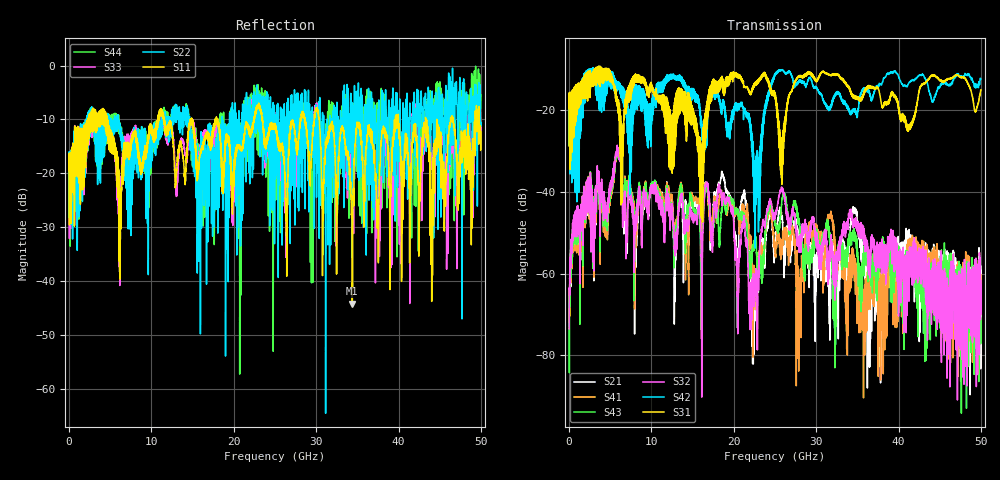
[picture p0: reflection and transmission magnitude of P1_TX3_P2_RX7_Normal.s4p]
!Keysight Technologies,N5225B,MY57041031,A.13.20.10
!Date: Friday, May 31, 2019 11:38:36
!Correction: S11(Full 4 Port(1,2,3,4))
!S12(Full 4 Port(1,2,3,4))
!S13(Full 4 Port(1,2,3,4))
!S14(Full 4 Port(1,2,3,4))
!S21(Full 4 Port(1,2,3,4))
!S22(Full 4 Port(1,2,3,4))
!S23(Full 4 Port(1,2,3,4))
!S24(Full 4 Port(1,2,3,4))
!S31(Full 4 Port(1,2,3,4))
!S32(Full 4 Port(1,2,3,4))
!S33(Full 4 Port(1,2,3,4))
!S34(Full 4 Port(1,2,3,4))
!S41(Full 4 Port(1,2,3,4))
!S42(Full 4 Port(1,2,3,4))
!S43(Full 4 Port(1,2,3,4))
!S44(Full 4 Port(1,2,3,4))
!S4P File: Measurements: <S11,S12,S13,S14>,
!<S21,S22,S23,S24>,
!<S31,S32,S33,S34>,
!<S41,S42,S43,S44>:
# Hz S  dB  R 50.0
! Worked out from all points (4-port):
!   5000 points, 10 MHz to 50 GHz, reference 50 ohm
!   strongest paths, dB at 10 MHz, 12.51 GHz, 25.01 GHz, 37.51 GHz, 50 GHz:
!     S31: -19.5, -27.1, -15.7, -14.5, -15.0
!     S42: -19.4, -12.2, -11.6, -14.0, -12.4
!     S32: -73.5, -42.8, -45.8, -55.0, -69.5
!     S43: -65.2, -42.9, -47.9, -57.0, -70.8
!     S41: -71.1, -40.8, -54.3, -69.6, -68.4
!     S21: -67.7, -41.2, -53.6, -64.7, -58.1
!   lowest |S11| = -44.2 dB at 34.39 GHz (marker M1), VSWR 1.01, Z = 50 + j0.617 ohm
!   |S11| at or under -10 dB: 4.66 GHz to 10.77 GHz (6.106 GHz wide, 79.2 % of centre); 23.49 GHz to 28.08 GHz (4.584 GHz wide, 17.8 % of centre); 30.37 GHz to 39.61 GHz (9.24 GHz wide, 26.4 % of centre)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
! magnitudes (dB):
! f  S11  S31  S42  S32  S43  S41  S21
! 10 MHz  -19.5  -19.5  -19.4  -73.5  -65.2  -71.1  -67.7
! 6.05 GHz  -29.4  -18.9  -14.4  -31.7  -31.4  -31.4  -31.4
! 21.24 GHz  -13.9  -14.2  -20.0  -46.3  -46.5  -45.4  -39.8
! 22.43 GHz  -10.2  -13.7  -35.1  -63.9  -52.8  -61.6  -72.5
! 24.37 GHz  -11.4  -13.8  -15.6  -42.7  -42.8  -44.0  -45.0
! 34.39 GHz  -44.2  -16.2  -20.0  -47.0  -51.0  -53.7  -44.7
! 50 GHz  -12.3  -15.0  -12.4  -69.5  -70.8  -68.4  -58.1
